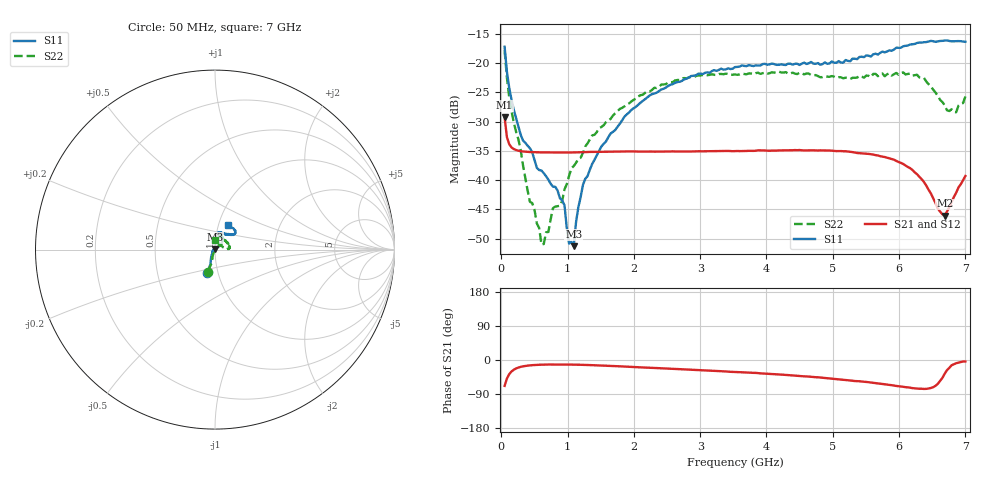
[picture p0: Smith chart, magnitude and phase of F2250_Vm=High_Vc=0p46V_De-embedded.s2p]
! Integrated Device Technology
! Corporate Headquarters
! 6024 Silver Creek Valley Road
! San Jose, CA 95138  USA
! Phone:  1-408-284-8200
! Toll Free:  1-800-223-1366
! Webpage:  http://www.idt.com/
! Timing and RF Division
! 515 Groton Road, Suite 102
! Westford, MA 01886-6024
! Device:  F2250
! Description: Voltage Variable RF Attenuator
! Frequency:  50.0 -  6000.00 MHz
! Package:  3x3 mm Thin QFN Plastic Package: 16 pin
! Ports:  2 RF, 3 DC
!  Pin  1  = GND
!  Pin  2  = NC
!  Pin  3  = RF1  = Port 1
!  Pin  4  = NC
!  Pin  5  = GND
!  Pin  6  = GND
!  Pin  7  = GND
!  Pin  8  = GND
!  Pin  9  = NC
!  Pin 10  = RF2  = Port 2
!  Pin 11  = NC
!  Pin 12  = GND
!  Pin 13  = GND
!  Pin 14  = VCNTRL
!  Pin 15  = VDD
!  Pin 16  = VMODE
! Vcntrl:  0.460 Volts
! Vmode:  +3.300 Volts
! Vdd:  +3.30  Volts
! Current:  1.264 mA
! Data:  The device was measured on a the F2250 evaluation board which has
!  individual transmission lines to the RF pins.  Data was collected
!  using a calibrated network analyzer.  The evaluation board was
!  de-embedded using a TRL calibration technique.
!  The reference plane is the edge of the package pin.
! Misc:  SN 10
!  Action Tracker AT0258
! Date Measured:  2014-11-26
! Date:  2015-10-15  MJV
! Note:
!  Integrated Device Technology supplies this data as a sample of measured
!  data at the package pin for this product.  Your particular data for this
!  product may vary.
!  Data was taken at 25 degrees C.
!  Integrated Device Technology reserves the right to change this data at anytime.
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# GHz S dB R 50
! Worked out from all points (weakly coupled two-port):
!   201 points, 50 MHz to 7 GHz, reference 50 ohm
!   highest |S21| = -29.27 dB at 50 MHz (marker M1); lowest = -46.1 dB at 6.687 GHz (marker M2)
!   lowest |S11| = -51.3 dB at 1.093 GHz (marker M3), VSWR 1.01, Z = 50 + j0.272 ohm
!   |S11| at or under -10 dB: start of sweep to end of sweep
!   |S22| runs from -51.0 to -17.8 dB; largest |S21 - S12| = 5.1e-05
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0.05  -17.17 -108.5  -29.27 -68.2  -29.27 -68.2  -17.80 -108.4
0.1195  -24.20 -111.9  -33.85 -37.4  -33.85 -37.4  -25.82 -106.4
0.29325  -32.26 -127.3  -35.04 -18.1  -35.04 -18.1  -34.91 -111.8
0.43225  -34.54 -145.2  -35.19 -14.1  -35.19 -14.2  -43.72 -143.8
0.50175  -36.61 -147.7  -35.22 -13.2  -35.22 -13.2  -45.12 -152.6
0.606  -38.36 -162.5  -35.25 -12.4  -35.25 -12.4  -51.00 164.0
0.71025  -39.93 -167.6  -35.27 -12.0  -35.27 -12.0  -48.86 105.2
0.77975  -41.11 176.4  -35.28 -11.9  -35.28 -11.9  -44.78 94.5
0.884  -43.08 165.3  -35.28 -11.9  -35.28 -11.9  -44.39 79.1
0.9535  -44.30 171.0  -35.29 -12.0  -35.28 -12.0  -41.57 78.6
1.023  -50.87 140.1  -35.28 -12.1  -35.27 -12.1  -39.24 63.7
1.0925  -51.30 89.2  -35.26 -12.2  -35.26 -12.2  -37.60 59.7
1.2315  -40.83 40.3  -35.21 -12.8  -35.21 -12.8  -35.32 45.2
1.6485  -32.02 41.1  -35.13 -15.6  -35.14 -15.6  -29.52 44.1
2.37825  -24.75 46.6  -35.11 -21.6  -35.10 -21.6  -24.07 45.5
3.525  -20.65 71.7  -35.04 -31.4  -35.04 -31.5  -21.92 68.5
4.7065  -20.06 72.0  -34.89 -44.9  -34.90 -44.8  -22.05 67.7
5.85325  -17.79 40.5  -36.29 -65.6  -36.29 -65.8  -21.72 19.1
6.3745  -16.40 40.9  -40.31 -76.3  -40.31 -76.4  -22.51 2.8
6.68725  -16.11 47.8  -46.07 -36.4  -46.06 -36.1  -27.19 24.8
6.861  -16.22 54.5  -42.15 -8.4  -42.11 -8.5  -28.38 58.4
7  -16.33 62.4  -39.29 -3.9  -39.25 -4.0  -25.69 87.4
